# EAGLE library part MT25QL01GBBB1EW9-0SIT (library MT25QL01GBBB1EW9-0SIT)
NOR Flash SPI FLASH NOR SLC 256MX4 WPDFN DDP Source: Datasheet
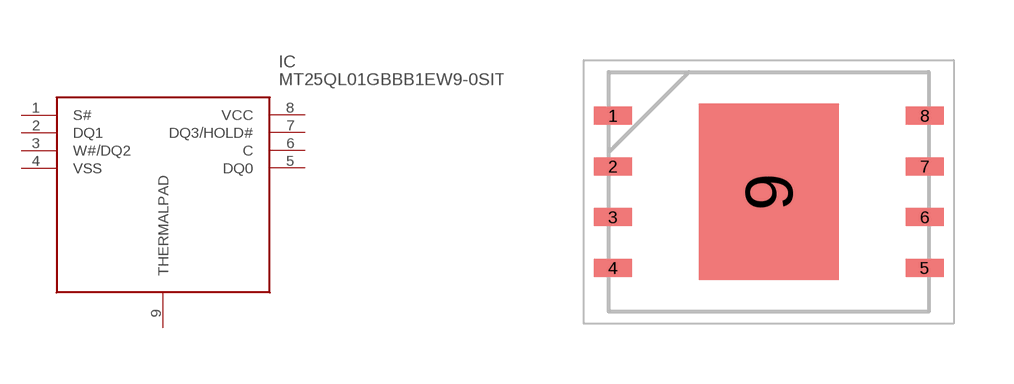
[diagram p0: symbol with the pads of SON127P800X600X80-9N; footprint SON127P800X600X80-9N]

Designator prefix IC

## MT25QL01GBBB1EW9-0SIT (Description: NOR Flash SPI FLASH NOR SLC 256MX4 WPDFN DDP; Height: 0.8mm; Manufacturer_Name: Micron; Manufacturer_Part_Number: MT25QL01GBBB1EW9-0SIT)  [SON127P800X600X80-9N]
1  S#
2  DQ1
3  W#/DQ2
4  VSS
5  DQ0
6  C
7  DQ3/HOLD#
8  VCC
9  THERMALPAD

## Footprint SON127P800X600X80-9N (pad centres in mm)
W-PDFN-8 (MLP8) 8MM X 6MM
smd 0.95 x 0.45: 1 -3.9,1.905; 2 -3.9,0.635; 3 -3.9,-0.635; 4 -3.9,-1.905; 5 3.9,-1.905; 6 3.9,-0.635; 7 3.9,0.635; 8 3.9,1.905
smd 3.5 x 4.4: 9 0,0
